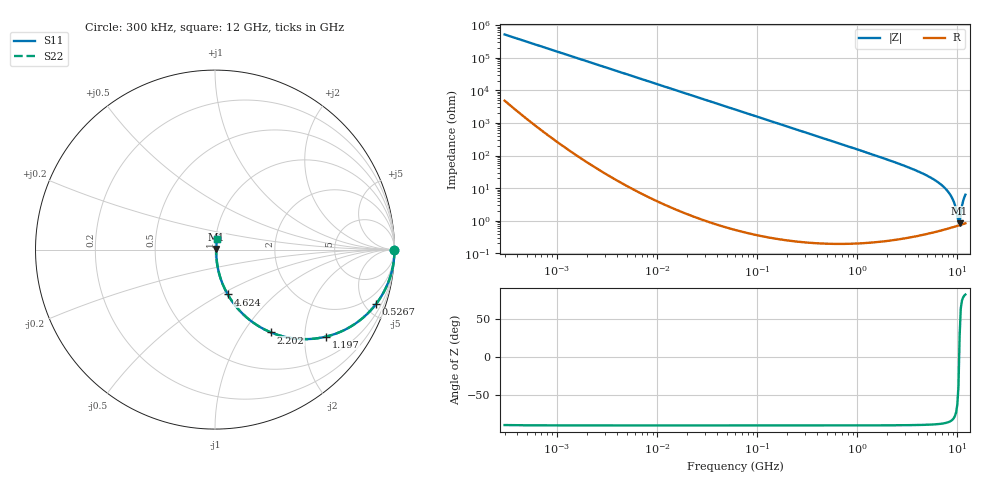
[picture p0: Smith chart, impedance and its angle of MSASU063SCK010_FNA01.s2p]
! MSASU063SCK010_FNA01  S-PARAMETER MODEL  ( Standard Model )
! Model Generated by TAIYO YUDEN Corporation (http://www.ty-top.com)
! Version 1.0
! TAIYO YUDEN Control No. 240819
! Copyright(c) 2024 TAIYO YUDEN CO.,LTD. All Rights Reserved.
! Product Description (link to TY-COMPAS)
! https://ds.yuden.co.jp/TYCOMPAS/or/detail?pn=MSASU063SCK010CFNA01&u=M
! Products Name : Multilayer Ceramic Capacitors
! Characteristics :
!  Capacitance : 1 [pF] , Rated Voltage : 50 [V] , TCC : CK / C0K
!  Case Size : 0.6 x 0.3 / 0.024 x 0.012 [mm/inch] , Thickness : 0.3 / 0.012 [mm/inch]
!  (Conditions: Temperature = 25 [degC] , DC Bias Voltage = 0 [V])
! External Node Assignments :
!  1  o---| |---o  2
! GND o---------o GND
! Frequency Range : 0.3MHz  -  12000MHz  [ 401 STEP ]
# MHZ S RI R 50
! Freq[MHz].  S11 Real  S11 Imag  S21 Real  S21 Imag  S12 Real  S12 Imag  S22 Real  S22 Imag
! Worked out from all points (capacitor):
!   401 points, 300 kHz to 12 GHz, reference 50 ohm
!   read as one part in series: C = 1.03 pF near 316.3 kHz
!   lowest |Z| = 826 mohm at 10.51 GHz (marker M1)
!   series resonance near 10.4 GHz, so ESL is about 230 pH
!   S11 on the Smith chart (normalised r, x): 300 kHz: open; 526.7 MHz: 1.00, -5.88; 1.197 GHz: 1.00, -2.56; 2.202 GHz: 1.00, -1.35; 4.624 GHz: 1.01, -0.54; 12 GHz: 1.02, +0.12
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0.3  1 -0.000193  1.84e-06 0.000193  1.84e-06 0.000193  1 -0.000193
1.769972  1 -0.00114  2.32e-06 0.00114  2.32e-06 0.00114  1 -0.00114
10.44266  1 -0.00673  4.69e-05 0.00673  4.69e-05 0.00673  1 -0.00673
60  0.9985 -0.0386  0.0015 0.0386  0.0015 0.0386  0.9985 -0.0386
159.8975  0.9895 -0.1019  0.0105 0.1019  0.0105 0.1019  0.9895 -0.1019
353.9943  0.9504 -0.2169  0.0496 0.2169  0.0496 0.2169  0.9504 -0.2169
526.7124  0.8962 -0.3047  0.1038 0.3047  0.1038 0.3047  0.8962 -0.3047
804.7407  0.786 -0.4096  0.214 0.4096  0.214 0.4096  0.786 -0.4096
1197.383  0.6207 -0.4844  0.3793 0.4844  0.3793 0.4844  0.6207 -0.4844
2088.533  0.3379 -0.4713  0.6621 0.4713  0.6621 0.4713  0.3379 -0.4713
2202.174  0.3128 -0.4618  0.6872 0.4618  0.6872 0.4618  0.3128 -0.4618
4623.766  0.0708 -0.2497  0.9292 0.2497  0.9292 0.2497  0.0708 -0.2497
6354.153  0.0274 -0.1487  0.9726 0.1487  0.9726 0.1487  0.0274 -0.1487
7854.144  0.0127 -0.084  0.9873 0.084  0.9873 0.084  0.0127 -0.084
8966.534  0.00824 -0.0444  0.9918 0.0444  0.9918 0.0444  0.00824 -0.0444
9454.42  0.00739 -0.0288  0.9926 0.0288  0.9926 0.0288  0.00739 -0.0288
9968.853  0.00706 -0.0132  0.9929 0.0132  0.9929 0.0132  0.00706 -0.0132
10236.47  0.00709 -0.00548  0.9929 0.00548  0.9929 0.00548  0.00709 -0.00548
10511.28  0.00726 0.00383  0.9927 -0.00383  0.9927 -0.00383  0.00726 0.00383
10793.46  0.00766 0.0153  0.9923 -0.0153  0.9923 -0.0153  0.00766 0.0153
11380.75  0.0093 0.0383  0.9907 -0.0383  0.9907 -0.0383  0.0093 0.0383
12000  0.012 0.0611  0.988 -0.0611  0.988 -0.0611  0.012 0.0611
